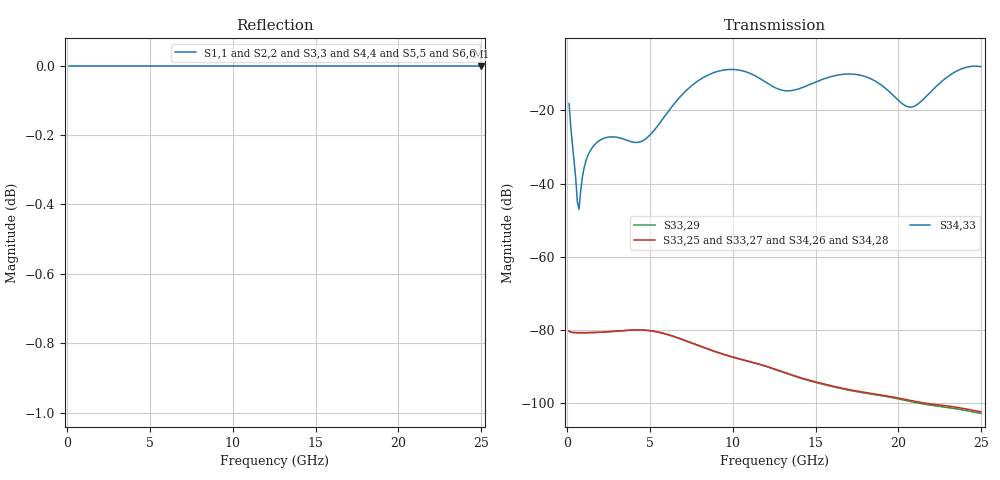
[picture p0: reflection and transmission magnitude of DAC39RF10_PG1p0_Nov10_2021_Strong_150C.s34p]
! Touchstone Ver. 1.0
! Number of ports is 34
# Hz	S	RI	R	50.000000
! SCATTERING PARAMETERS  :
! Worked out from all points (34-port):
!   250 points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, 100 MHz to 25 GHz, reference 50 ohm
!   strongest paths, dB at 100 MHz, 6.3 GHz, 12.6 GHz, 18.8 GHz, 25 GHz:
!     S34,33: -18.2, -19.1, -13.9, -12.5, -8.1
!     S33,25: -80.4, -81.6, -90.8, -97.6, -102.4
!     S33,27: -80.4, -81.6, -90.8, -97.7, -102.5
!     S33,29: -80.4, -81.6, -90.9, -97.8, -102.8
!     S34,26: -80.4, -81.6, -90.9, -97.7, -102.6
!     S34,28: -80.4, -81.6, -90.9, -97.8, -102.8
!   lowest |S11| = 0.0 dB at 25 GHz (marker M1)
!   |S11| at or under -10 dB: nowhere
